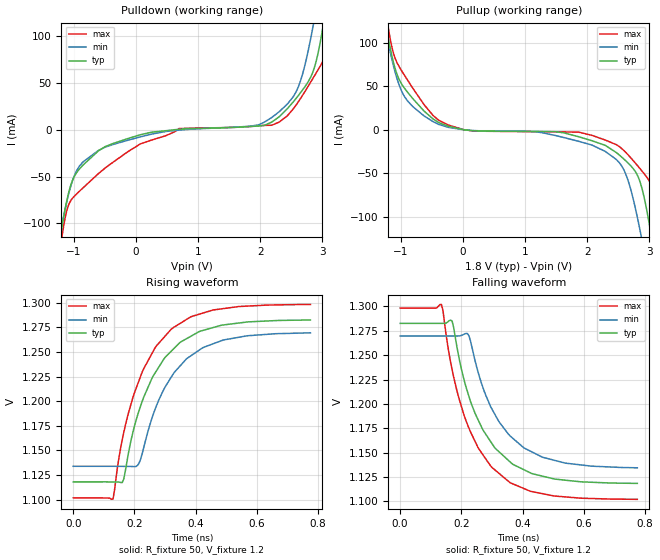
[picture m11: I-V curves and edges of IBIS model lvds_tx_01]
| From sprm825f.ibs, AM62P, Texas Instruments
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[Model] lvds_tx_01
Model_type Output
C_comp 1.451p 1.479p 1.402p
Vmeas = 1.2
Vref = 1.2V
Rref = 50
Cref = 0.5pF
[Model Spec]
[Temperature Range]  40 150 -40
[Voltage Range] 1.8 1.62 1.98
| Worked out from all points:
|   slope of the pulldown table from 0 to 0.27 V, typ, clamps not added: 62.8 ohm
|   slope of the pullup table from 0 to 0.27 V, typ, clamps not added: 160 ohm
|   rising waveform, R_fixture 50, V_fixture 1.2: 20-80 % time 134ps typ, 131ps min, 131ps max; typ from 1.12 V to 1.28 V
|   falling waveform, R_fixture 50, V_fixture 1.2: 20-80 % time 131ps typ, 134ps min, 129ps max; typ from 1.28 V to 1.12 V
[Pulldown]
-1.715V   -358.4mA   -310.5mA   -423.2mA
-1.208V   -111mA     -107mA     -122mA
-1.002V   -51.14mA   -50.85mA   -71.71mA
-494mV    -17.98mA   -18.54mA   -40.83mA
690.4mV   474uA      -435.5uA   1.234mA
1.97V     4.003mA    5.129mA    4.182mA
2.308V    13.98mA    19.41mA    8.266mA
2.62V     37.11mA    46.95mA    30.47mA
2.858V    63.6mA     113.1mA    55.89mA
3.006V    108.2mA    169.3mA    72.77mA
3.175V    183.2mA    238.4mA    115.4mA
3.514V    352mA      380.5mA    305.9mA
[Pullup]
-1.714V   352mA      304.8mA    416.6mA
-1.259V   130mA      120.6mA    145.9mA
-1.206V   108.2mA    101.9mA    120.1mA
-894.3mV  43.58mA    33.55mA    57.67mA
-228.1mV  3.872mA    2.691mA    5.3mA
1.268V    -2.008mA   -3.301mA   -2.291mA
2.474V    -26.38mA   -34.44mA   -17.27mA
2.669V    -38.97mA   -60.46mA   -29.61mA
2.86V     -61.59mA   -118.3mA   -45.42mA
3.034V    -122.1mA   -185.4mA   -63.83mA
3.203V    -201mA     -255.1mA   -126.9mA
3.515V    -358.4mA   -386.1mA   -310.8mA
[Ramp]
dV/dt_r .099/134.293p .081/131.639p .118/131.436p
dV/dt_f .099/131.621p .081/135.062p .118/129.186p
[Rising Waveform]
R_fixture = 50
V_fixture = 1.2
V_fixture_min = 1.202
V_fixture_max = 1.2
0s        1.118V     1.134V     1.102V
130ps     1.118V     1.134V     1.101V
165ps     1.121V     1.134V     1.168V
200ps     1.175V     1.134V     1.209V
220ps     1.195V     1.141V     1.225V
260ps     1.225V     1.185V     1.25V
320ps     1.251V     1.224V     1.273V
370ps     1.263V     1.243V     1.283V
490ps     1.277V     1.262V     1.294V
775ps     1.282V     1.269V     1.298V
[Falling Waveform]
R_fixture = 50
V_fixture = 1.2
V_fixture_min = 1.202
V_fixture_max = 1.2
0s        1.283V     1.27V      1.298V
135ps     1.283V     1.27V      1.302V
170ps     1.285V     1.27V      1.235V
215ps     1.218V     1.272V     1.183V
225ps     1.207V     1.27V      1.175V
260ps     1.18V      1.227V     1.153V
295ps     1.162V     1.198V     1.137V
355ps     1.142V     1.169V     1.12V
465ps     1.126V     1.145V     1.108V
775ps     1.118V     1.134V     1.102V
